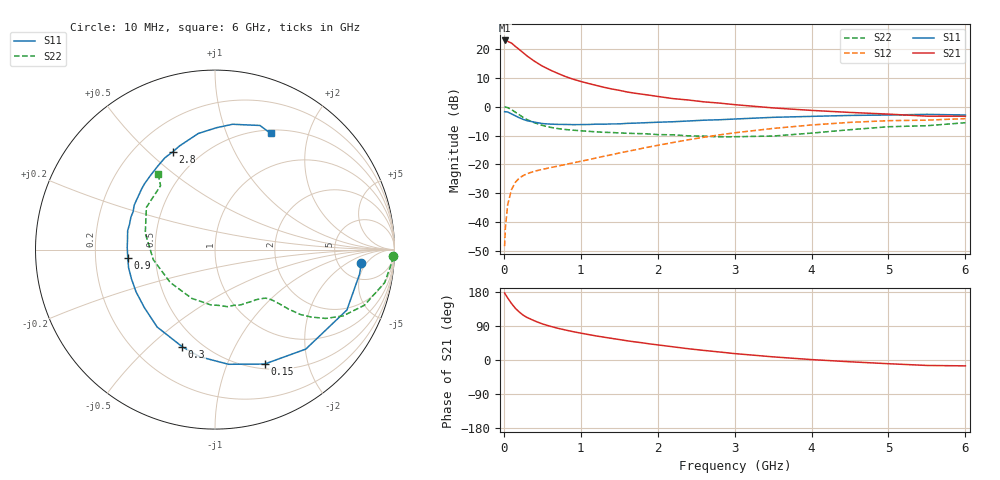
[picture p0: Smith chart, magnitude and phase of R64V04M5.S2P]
! SIEMENS Small Signal Semiconductors
! BFR193
! Si NPN RF Bipolar Junction Transistor in SOT23
! VCE = 4 V  IC = 4.5 mA
! Common Emitter S-Parameters:  May  1996
# GHz  S  MA  R  50
!  f  S11  S21  S12  S22
! GHz  MAG  ANG  MAG  ANG  MAG  ANG  MAG  ANG
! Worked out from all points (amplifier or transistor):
!   36 points, 10 MHz to 6 GHz, reference 50 ohm
!   highest |S21| = 23.0 dB at 10 MHz (marker M1)
!   |S21| within 3 dB of that: start of sweep to 194.2 MHz
!   unconditionally stable (mu >= 1): 933.7 MHz to 1.992 GHz
!   at 250 MHz: K = 0.40, MSG = 21.3 dB, |S12| = -23.9 dB
!   at 1.4 GHz: K = 1.07, MAG = 9.8 dB, |S12| = -16.7 dB
!   at 6 GHz: K = 0.97, MSG = 0.4 dB, |S12| = -4.1 dB
!   S11 on the Smith chart (normalised r, x): 10 MHz: 8.40, -3.72; 150 MHz: 0.56, -1.37; 300 MHz: 0.40, -0.64; 900 MHz: 0.34, -0.04; 2.8 GHz: 0.36, +0.60; 6 GHz: 0.54, +1.45
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0.01  0.8192 -5.1  14.1 176.9  0.0038 86.6  0.9938 -2.2
0.02  0.8169 -9.7  13.95 173.2  0.0079 81.7  0.9858 -4.6
0.05  0.8082 -24.6  13.61 163.7  0.02 78.3  0.963 -11.0
0.1  0.7505 -47.6  12.68 149.0  0.0365 67.2  0.8887 -20.4
0.15  0.6949 -66.6  11.1 136.4  0.0489 59.1  0.8031 -27.4
0.2  0.6433 -83.3  9.842 126.7  0.0575 54.2  0.7257 -31.9
0.25  0.6033 -98.0  8.662 118.5  0.0636 49.9  0.6529 -35.1
0.3  0.5711 -108.7  7.622 112.4  0.0686 47.9  0.5989 -37.2
0.4  0.5384 -126.8  6.124 103.2  0.076 45.6  0.5254 -39.0
0.5  0.5092 -140.7  5.066 95.3  0.0817 45.7  0.4739 -40.0
0.6  0.4988 -151.9  4.345 89.2  0.0873 47.1  0.4396 -40.9
0.7  0.4931 -160.7  3.79 83.8  0.093 48.3  0.4175 -41.8
0.9  0.4882 -174.7  3 74.8  0.1059 51.3  0.391 -43.8
1.1  0.491 173.1  2.528 67.2  0.1202 54.5  0.3736 -47.4
1.3  0.4966 163.5  2.173 60.3  0.1379 56.8  0.3594 -51.3
1.6  0.5135 151.3  1.802 50.8  0.1671 58.8  0.3459 -58.8
2.2  0.548 130.9  1.381 34.8  0.239 58.0  0.3251 -77.9
2.8  0.5931 113.5  1.155 21.2  0.3237 52.1  0.2995 -104.7
3.5  0.6536 98.2  0.952 8.3  0.4193 41.4  0.3094 -143.7
4.5  0.7052 82.0  0.795 -4.7  0.5346 24.2  0.3988 166.9
5.5  0.7356 70.1  0.685 -14.4  0.5838 6.7  0.4678 130.4
6  0.7176 64.4  0.685 -15.5  0.621 1.7  0.527 127.0
